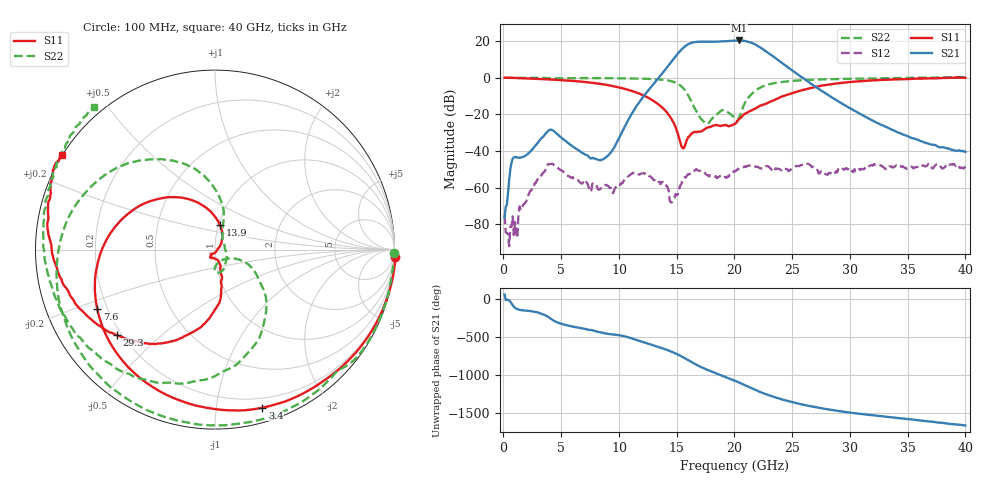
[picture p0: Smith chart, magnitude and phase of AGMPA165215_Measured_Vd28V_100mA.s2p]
! TFN Cal with 50ohm delay
! AG06_M040_Carrier1_n1p71_0_28_103mA
!Keysight Technologies,N5245B,MY58421923,A.15.75.19
!Date: Tuesday, February 21, 2023 09:01:13
!Correction: S11(C  2-Port  )
!S21(C  2-Port  )
!S12(C  2-Port  )
!S22(C  2-Port  )
!S2P File: Measurements: S11, S21, S12, S22:
# Hz S  dB  R 50
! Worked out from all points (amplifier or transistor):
!   400 points, 100 MHz to 40 GHz, reference 50 ohm
!   highest |S21| = 20.4 dB at 20.4 GHz (marker M1)
!   |S21| within 3 dB of that: 15.76 GHz to 22.03 GHz (6.262 GHz wide, 33.1 % of centre)
!   unconditionally stable (mu >= 1): 599.8 MHz to 35.36 GHz; 35.59 GHz to 35.78 GHz
!   at 6.7 GHz: K = 633.61, MAG = -22.5 dB, |S12| = -57.6 dB
!   at 20.1 GHz: K = 16.60, MAG = 20.4 dB, |S12| = -50.8 dB
!   at 40 GHz: K = 7.22, MSG = 3.8 dB, |S12| = -48.0 dB
!   S11 on the Smith chart (normalised r, x): 100 MHz: -7, -49; 3.4 GHz: 0.12, -1.34; 7.6 GHz: 0.16, -0.23; 13.9 GHz: 1.02, +0.28; 29.3 GHz: 0.18, -0.36; 40 GHz: -0.00, +0.28
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1e8  0.05 -2.3  -76.34 63.5  -75.27 34.9  -0.03 -1.0
3.4e9  -0.73 -73.3  -32.44 163.6  -52.20 -85.4  -0.07 -36.5
6.8e9  -2.14 -138.4  -41.03 -22.6  -57.83 16.2  -0.18 -71.1
7.6e9  -2.68 -153.2  -44.11 -43.8  -61.72 4.2  -0.19 -80.2
1.34e10  -14.46 91.4  -0.31 92.9  -56.85 132.0  -0.88 -166.5
1.39e10  -17.17 78.2  3.60 67.8  -57.19 122.9  -1.18 -179.4
1.48e10  -25.46 48.0  10.86 14.7  -65.78 174.8  -2.41 149.4
1.54e10  -37.23 5.7  15.31 -30.3  -58.05 -160.7  -4.66 120.6
1.62e10  -31.12 -119.3  18.95 -100.3  -52.38 174.8  -12.00 80.3
1.68e10  -29.51 -133.4  19.67 -149.5  -50.57 147.9  -19.30 66.6
1.73e10  -28.68 -125.2  19.74 174.6  -51.53 130.8  -23.64 44.7
1.87e10  -26.20 -119.6  19.80 88.2  -53.96 138.8  -18.76 -64.3
1.93e10  -25.91 -109.9  20.03 52.7  -54.83 134.5  -18.30 -88.8
2.01e10  -24.94 -79.1  20.33 3.8  -50.82 139.6  -22.61 -74.6
2.04e10  -22.61 -72.3  20.41 -15.7  -49.80 135.0  -21.79 -39.0
2.13e10  -18.32 -75.3  19.52 -78.1  -47.98 117.5  -10.19 -35.9
2.23e10  -15.09 -78.9  16.32 -145.0  -49.56 104.8  -5.14 -63.7
2.37e10  -11.48 -83.1  10.09 140.3  -49.84 95.7  -2.69 -96.4
2.67e10  -5.48 -111.7  -3.51 28.4  -48.88 64.2  -1.12 -139.3
2.93e10  -2.79 -139.0  -14.06 -37.4  -50.01 80.8  -0.63 -164.4
3.34e10  -1.03 -173.7  -27.67 -112.5  -48.46 68.2  -0.24 165.7
4e10  0.03 148.5  -40.49 138.1  -48.00 32.3  0.35 130.3
